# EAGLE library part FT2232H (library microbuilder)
FTDI 2232H - Dual High-Speed USB to UART/FIFO
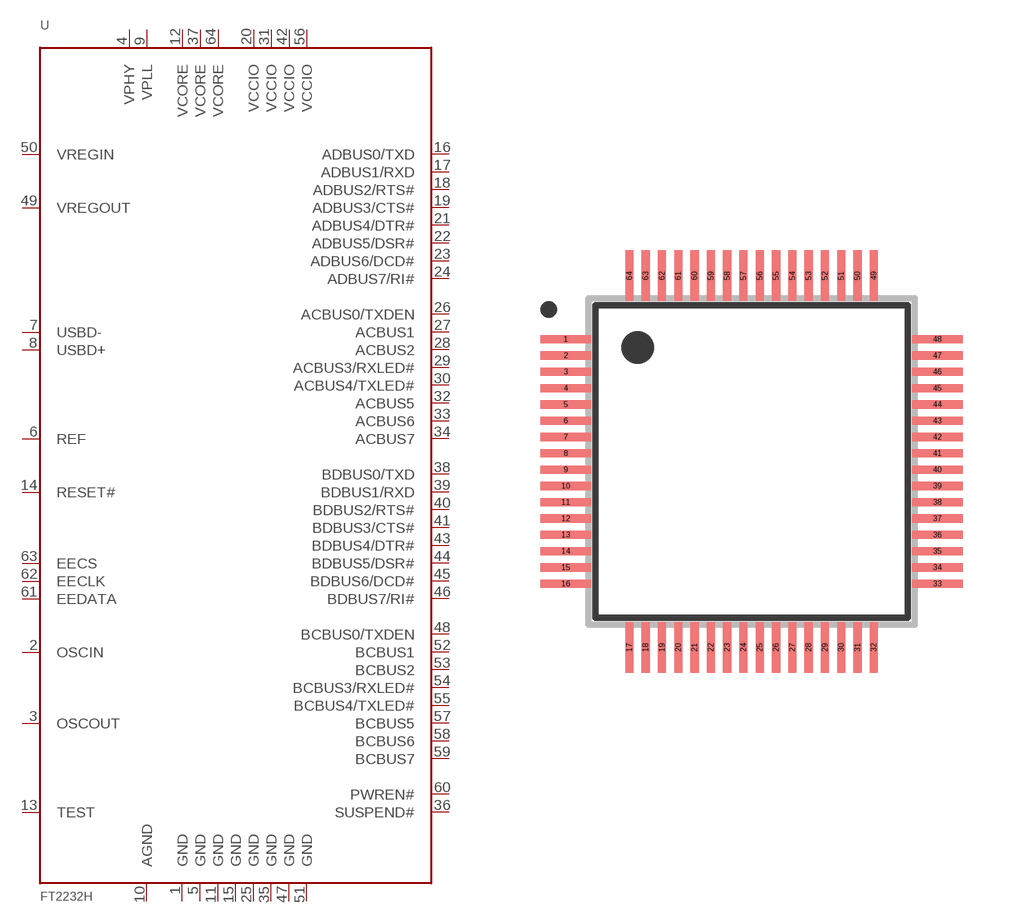
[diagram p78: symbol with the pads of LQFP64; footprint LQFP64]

Designator prefix U

## FT2232H  [LQFP64]
1  GND
2  OSCIN
3  OSCOUT
4  VPHY
5  GND
6  REF
7  USBD-
8  USBD+
9  VPLL
10  AGND
11  GND
12  VCORE
13  TEST
14  RESET#
15  GND
16  ADBUS0/TXD
17  ADBUS1/RXD
18  ADBUS2/RTS#
19  ADBUS3/CTS#
20  VCCIO
21  ADBUS4/DTR#
22  ADBUS5/DSR#
23  ADBUS6/DCD#
24  ADBUS7/RI#
25  GND
26  ACBUS0/TXDEN
27  ACBUS1
28  ACBUS2
29  ACBUS3/RXLED#
30  ACBUS4/TXLED#
31  VCCIO
32  ACBUS5
33  ACBUS6
34  ACBUS7
35  GND
36  SUSPEND#
37  VCORE
38  BDBUS0/TXD
39  BDBUS1/RXD
40  BDBUS2/RTS#
41  BDBUS3/CTS#
42  VCCIO
43  BDBUS4/DTR#
44  BDBUS5/DSR#
45  BDBUS6/DCD#
46  BDBUS7/RI#
47  GND
48  BCBUS0/TXDEN
49  VREGOUT
50  VREGIN
51  GND
52  BCBUS1
53  BCBUS2
54  BCBUS3/RXLED#
55  BCBUS4/TXLED#
56  VCCIO
57  BCBUS5
58  BCBUS6
59  BCBUS7
60  PWREN#
61  EEDATA
62  EECLK
63  EECS
64  VCORE

## Footprint LQFP64 (pad centres in mm)
smd 1.55 x 0.25: 1 -5.7,3.75; 2 -5.7,3.25; 3 -5.7,2.75; 4 -5.7,2.25; 5 -5.7,1.75; 6 -5.7,1.25; 7 -5.7,0.75; 8 -5.7,0.25; 9 -5.7,-0.25; 10 -5.7,-0.75; 11 -5.7,-1.25; 12 -5.7,-1.75; 13 -5.7,-2.25; 14 -5.7,-2.75; 15 -5.7,-3.25; 16 -5.7,-3.75; 33 5.7,-3.75; 34 5.7,-3.25; 35 5.7,-2.75; 36 5.7,-2.25; 37 5.7,-1.75; 38 5.7,-1.25; 39 5.7,-0.75; 40 5.7,-0.25; 41 5.7,0.25; 42 5.7,0.75; 43 5.7,1.25; 44 5.7,1.75; 45 5.7,2.25; 46 5.7,2.75; 47 5.7,3.25; 48 5.7,3.75
smd 0.25 x 1.55: 17 -3.75,-5.7; 18 -3.25,-5.7; 19 -2.75,-5.7; 20 -2.25,-5.7; 21 -1.75,-5.7; 22 -1.25,-5.7; 23 -0.75,-5.7; 24 -0.25,-5.7; 25 0.25,-5.7; 26 0.75,-5.7; 27 1.25,-5.7; 28 1.75,-5.7; 29 2.25,-5.7; 30 2.75,-5.7; 31 3.25,-5.7; 32 3.75,-5.7; 49 3.75,5.7; 50 3.25,5.7; 51 2.75,5.7; 52 2.25,5.7; 53 1.75,5.7; 54 1.25,5.7; 55 0.75,5.7; 56 0.25,5.7; 57 -0.25,5.7; 58 -0.75,5.7; 59 -1.25,5.7; 60 -1.75,5.7; 61 -2.25,5.7; 62 -2.75,5.7; 63 -3.25,5.7; 64 -3.75,5.7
